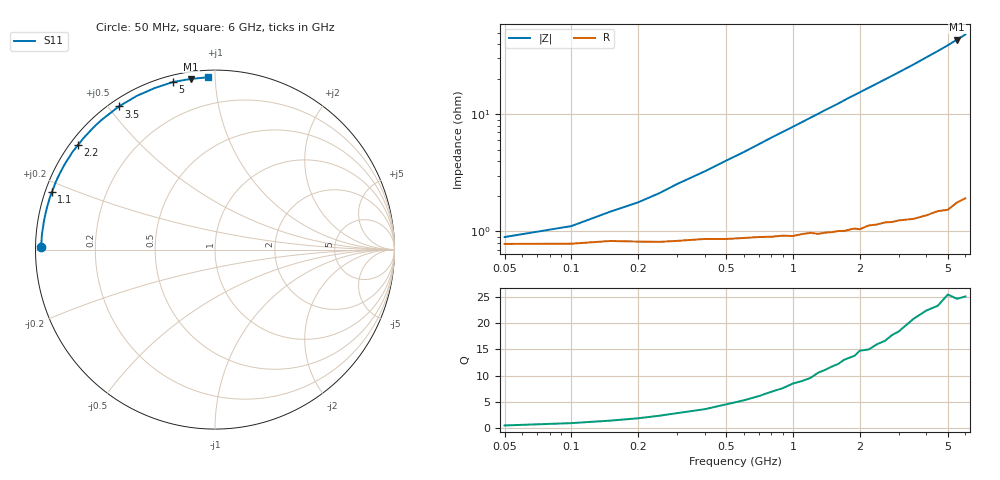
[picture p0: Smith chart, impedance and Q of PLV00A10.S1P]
! Infineon Technologies  Discrete & RF Semiconductors
! BAR 64-04W /-05W /-06W
! Si PIN Diode in SOT323
! IF = 100 mA
! S-Parameters:  October  2008
# GHz  S  MA  R  50
!  f  S11
! GHz  MAG  ANG
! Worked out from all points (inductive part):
!   34 points, 50 MHz to 6 GHz, reference 50 ohm
!   read as one part to ground: L = 1.25 nH near 400 MHz
!   highest Q = 25 at 5.5 GHz (marker M1), where L = 1.26 nH
!   S11 on the Smith chart (normalised r, x): 50 MHz: 0.02, +0.01; 1.1 GHz: 0.02, +0.17; 2.2 GHz: 0.02, +0.34; 3.5 GHz: 0.03, +0.53; 5 GHz: 0.03, +0.78; 6 GHz: 0.04, +0.96
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0.05  0.9692 179.0
0.1  0.9691 178.2
0.15  0.9674 177.2
0.25  0.968 175.5
0.3  0.9674 174.5
0.4  0.9662 172.8
0.5  0.9663 171.0
0.6  0.9657 169.3
0.8  0.9651 165.7
1  0.9649 162.3
1.1  0.9637 160.6
1.3  0.964 157.2
1.4  0.9634 155.5
1.6  0.9627 152.3
1.8  0.9622 148.9
1.9  0.9617 147.4
2  0.9626 145.8
2.2  0.9604 142.7
2.4  0.9604 139.7
2.6  0.9596 136.7
2.8  0.9601 133.8
3  0.9597 130.9
3.5  0.9609 123.9
4  0.9609 116.9
4.5  0.9605 110.5
5  0.9626 104.2
5.5  0.9605 98.0
6  0.9609 92.2
